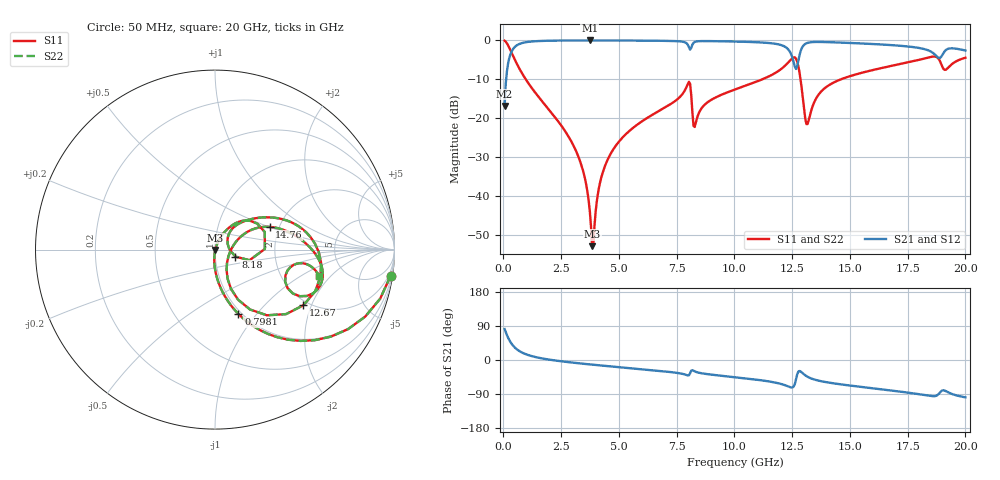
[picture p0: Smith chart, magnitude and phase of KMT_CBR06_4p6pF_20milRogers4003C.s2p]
! Data measured by Modelithics Inc. support@modelithics.com 813-866-6335
! KEMET CBR0603 4.6pF, Pad Width= 0.851mm, Pad Length= 0.64mm, Pad Gap= 0.62mm, 20mil Rogers 4003C substrate Data, January 2022
# hz S ma R 50
! 2 Port Network Data from SP1.SP block
! freq  magS11  angS11  magS21  angS21  magS12  angS12  magS22  angS22
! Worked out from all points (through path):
!   401 points, 50 MHz to 20 GHz, reference 50 ohm
!   highest |S21| = -0.02 dB at 3.741 GHz (marker M1); lowest = -16.8 dB at 50 MHz (marker M2)
!   group delay of S21, straight-line fit = 15.8 ps
!   lowest |S11| = -52.8 dB at 3.841 GHz (marker M3), VSWR 1.00, Z = 50.2 - j0.157 ohm
!   |S11| at or under -10 dB: 967.1 MHz to 11.2 GHz (10.23 GHz wide, 168 % of centre); 12.86 GHz to 14.61 GHz (1.744 GHz wide, 12.7 % of centre)
!   |S22| runs from -52.8 to -0.1 dB; largest |S21 - S12| = 0
!   S11 on the Smith chart (normalised r, x): 50 MHz: 1, -13; 798.1 MHz: 0.97, -0.81; 8.18 GHz: 1.25, -0.10; 12.67 GHz: 1.87, -1.75; 14.76 GHz: 1.78, +0.51; 20 GHz: 3.24, -1.50
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5e7  0.9895 -8.5  0.1442 81.5  0.1442 81.5  0.9895 -8.5
2.99375e8  0.7513 -42.2  0.6591 47.7  0.6591 47.7  0.7513 -42.2
7.98125e8  0.381 -70.0  0.9235 19.8  0.9235 19.8  0.381 -70.0
3.391625e9  0.02416 -95.1  0.9977 -9.5  0.9977 -9.5  0.02416 -95.1
3.74075e9  0.006358 -83.8  0.9979 -11.6  0.9979 -11.6  0.006358 -83.8
3.8405e9  0.002294 -43.0  0.9979 -12.2  0.9979 -12.2  0.002294 -43.0
4.189625e9  0.01532 68.0  0.9977 -14.3  0.9977 -14.3  0.01532 68.0
4.6385e9  0.03502 69.6  0.997 -16.9  0.997 -16.9  0.03502 69.6
6.73325e9  0.1244 59.8  0.9887 -28.6  0.9887 -28.6  0.1244 59.8
7.980125e9  0.2765 31.6  0.8804 -40.7  0.8804 -40.7  0.2765 31.6
8.179625e9  0.1197 -18.9  0.8811 -27.0  0.8811 -27.0  0.1197 -18.9
8.32925e9  0.08822 37.8  0.9648 -31.2  0.9648 -31.2  0.08822 37.8
1.0025e10  0.2345 43.3  0.9664 -45.4  0.9664 -45.4  0.2345 43.3
1.211975e10  0.4528 19.5  0.8496 -65.1  0.8496 -65.1  0.4528 19.5
1.266838e10  0.5822 -32.2  0.43 -50.5  0.43 -50.5  0.5822 -32.2
1.291775e10  0.2361 -67.8  0.7968 -32.9  0.7968 -32.9  0.2361 -67.8
1.311725e10  0.08426 -28.3  0.9176 -42.5  0.9176 -42.5  0.08426 -28.3
1.336662e10  0.1377 23.5  0.9508 -49.7  0.9508 -49.7  0.1377 23.5
1.476312e10  0.3292 22.6  0.9331 -65.5  0.9331 -65.5  0.3292 22.6
1.670825e10  0.4647 8.7  0.8735 -79.9  0.8735 -79.9  0.4647 8.7
1.885288e10  0.5733 -26.8  0.5945 -89.1  0.5945 -89.1  0.5733 -26.8
2e10  0.5994 -14.4  0.7418 -98.6  0.7418 -98.6  0.5994 -14.4
